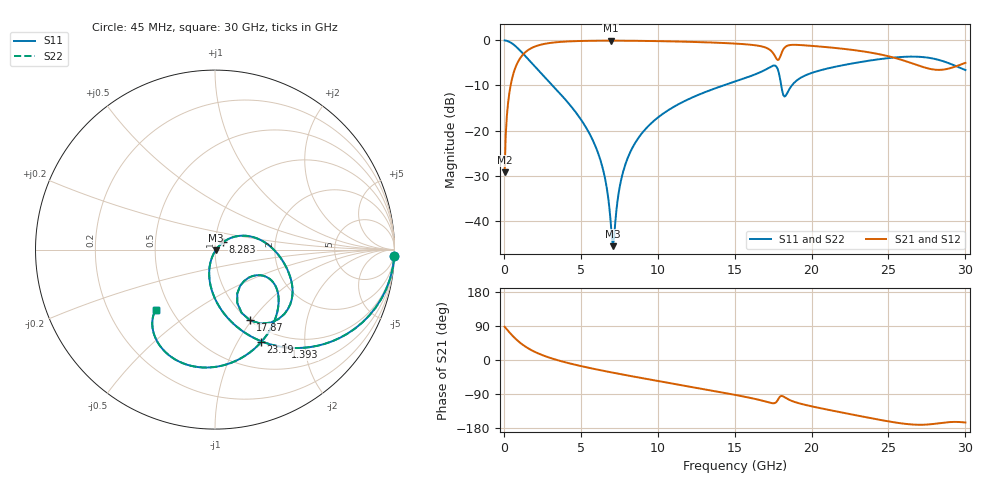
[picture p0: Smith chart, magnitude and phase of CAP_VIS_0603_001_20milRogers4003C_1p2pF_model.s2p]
! S-parameter model data by Modelithics Inc.  support@modelithics.com  813-866-6335  Tampa FL USA
! S-Parameter data specifications:
! Substrate: 20-mil Rogers 4003C, substrate thickness, H=0.508mm, Dielectric constant, Er=3.75
! PCB Mounting Pad Footprint: Pad width, PadW=0.90mm , Pad length, PadL=1.00mm , Pad gap, PadG (edge-to-edge)=1.00mm , Reference planes=3.0mm apart
! Created Wed Nov 18 13:17:57 2015
# hz S ma R 50
! 2 Port Network Data from SP1.SP block
! freq  magS11  angS11  magS21  angS21  magS12  angS12  magS22  angS22
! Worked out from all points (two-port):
!   401 points, 45 MHz to 30 GHz, reference 50 ohm
!   highest |S21| = -0.05 dB at 6.935 GHz (marker M1); lowest = -29.3 dB at 45 MHz (marker M2)
!   |S21| within 3 dB of the highest: 1.261 GHz to 17.54 GHz (16.28 GHz wide, 173 % of centre); 18.02 GHz to 24.39 GHz (6.367 GHz wide, 30 % of centre)
!   lowest |S11| = -45.7 dB at 7.084 GHz (marker M3), VSWR 1.01, Z = 50.4 - j0.319 ohm
!   |S11| at or under -10 dB: 3.165 GHz to 14.26 GHz (11.1 GHz wide, 127 % of centre); 18.03 GHz to 18.72 GHz (689.6 MHz wide, 3.75 % of centre)
!   |S22| runs from -45.7 to 0.0 dB; largest |S21 - S12| = 0
!   S11 on the Smith chart (normalised r, x): 45 MHz: 1, -52; 1.393 GHz: 0.82, -1.63; 8.283 GHz: 1.09, +0.09; 17.87 GHz: 1.00, -0.98; 23.19 GHz: 0.82, -1.26; 30 GHz: 0.42, -0.36
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4.5e7  0.9994 -2.2  0.03438 87.8  0.03438 87.8  0.9994 -2.2
2.696625e8  0.9793 -12.9  0.2022 77.0  0.2022 77.0  0.9793 -12.9
4.94325e8  0.9347 -23.1  0.3548 66.8  0.3548 66.8  0.9347 -23.1
1.392975e9  0.67 -54.4  0.7404 35.5  0.7404 35.5  0.67 -54.4
2.815838e9  0.366 -81.4  0.9274 8.2  0.9274 8.2  0.366 -81.4
5.062462e9  0.1284 -104.6  0.987 -16.5  0.987 -16.5  0.1284 -104.6
6.33555e9  0.04329 -111.0  0.9937 -27.5  0.9937 -27.5  0.04329 -111.0
6.709988e9  0.02175 -107.1  0.9942 -30.5  0.9942 -30.5  0.02175 -107.1
6.93465e9  0.009984 -91.3  0.9942 -32.3  0.9942 -32.3  0.009984 -91.3
7.084425e9  0.005212 -37.4  0.9942 -33.4  0.9942 -33.4  0.005212 -37.4
7.608638e9  0.02781 41.2  0.9935 -37.5  0.9935 -37.5  0.02781 41.2
8.282625e9  0.06103 42.0  0.9917 -42.6  0.9917 -42.6  0.06103 42.0
1.007992e10  0.1425 31.5  0.9823 -55.8  0.9823 -55.8  0.1425 31.5
1.50225e10  0.35 -4.0  0.9229 -92.0  0.9229 -92.0  0.35 -4.0
1.726912e10  0.5022 -31.0  0.7912 -112.4  0.7912 -112.4  0.5022 -31.0
1.786822e10  0.4394 -63.7  0.6129 -101.1  0.6129 -101.1  0.4394 -63.7
1.831755e10  0.2436 -40.2  0.8534 -100.0  0.8534 -100.0  0.2436 -40.2
2.003996e10  0.4379 -36.2  0.8696 -122.6  0.8696 -122.6  0.4379 -36.2
2.318524e10  0.576 -63.5  0.7634 -148.2  0.7634 -148.2  0.576 -63.5
2.505742e10  0.6383 -82.4  0.6636 -162.4  0.6636 -162.4  0.6383 -82.4
2.812781e10  0.6169 -119.9  0.4719 -167.8  0.4719 -167.8  0.6169 -119.9
3e10  0.4689 -134.5  0.5637 -165.0  0.5637 -165.0  0.4689 -134.5
